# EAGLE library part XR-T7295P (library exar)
DS3/Sonet STS-1 LINE RECEIVER
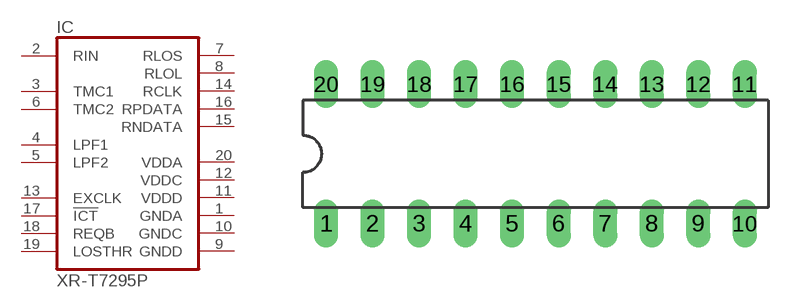
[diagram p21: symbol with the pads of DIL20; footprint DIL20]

Designator prefix IC

## XR-T7295P (OC_FARNELL: unknown; OC_NEWARK: unknown)  [DIL20]
1  GNDA  pwr
2  RIN  in
3  TMC1  in
4  LPF1  in
5  LPF2  in
6  TMC2  in
7  RLOS  out
8  RLOL  out
9  GNDD  pwr
10  GNDC  pwr
11  VDDD  pwr
12  VDDC  pwr
13  EXCLK  in
14  RCLK  out
15  RNDATA  out
16  RPDATA  out
17  !ICT  in
18  REQB  in
19  LOSTHR  in
20  VDDA  pwr

## Footprint DIL20 (pad centres in mm)
Dual In Line Package
drill 0.813 long: 1 -11.43,-3.81; 2 -8.89,-3.81; 3 -6.35,-3.81; 4 -3.81,-3.81; 5 -1.27,-3.81; 6 1.27,-3.81; 7 3.81,-3.81; 8 6.35,-3.81; 9 8.89,-3.81; 10 11.43,-3.81; 11 11.43,3.81; 12 8.89,3.81; 13 6.35,3.81; 14 3.81,3.81; 15 1.27,3.81; 16 -1.27,3.81; 17 -3.81,3.81; 18 -6.35,3.81; 19 -8.89,3.81; 20 -11.43,3.81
